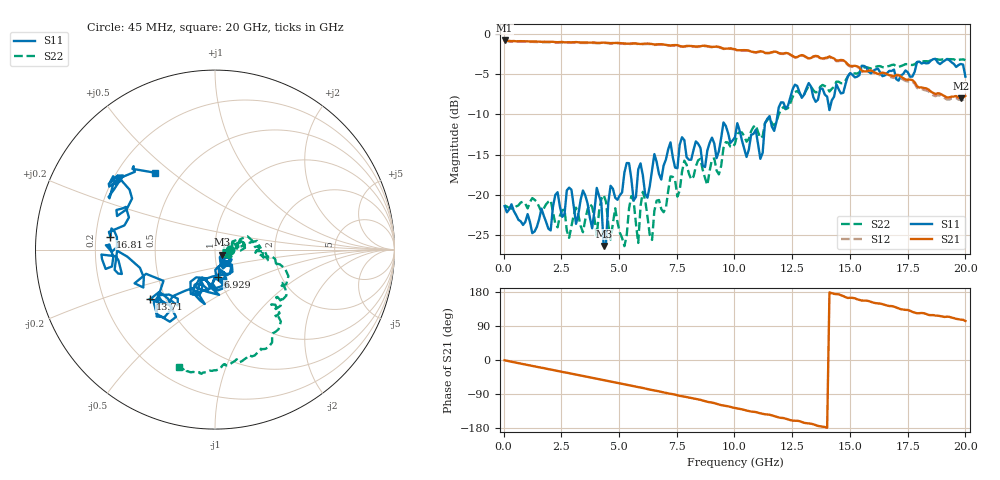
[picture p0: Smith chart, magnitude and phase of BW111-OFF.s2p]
!  2-Port S-parameters saved by WinCal
! VAR MeasName=S-Parameters (CALIBRATED_DATA) read from VNA (E8364A)
! VAR MeasDate=10/28/2010 3:35:15 PM
! VAR NAME=5-1you 2
! VAR FILENAME=5-1you 2.s2p
! VAR DATE=10/28/2010 3:35:15 PM
! VAR PHYS_PORTS=1,2
# Hz S RI R 50
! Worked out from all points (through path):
!   201 points, 45 MHz to 20 GHz, reference 50 ohm
!   highest |S21| = -0.83 dB at 45 MHz (marker M1); lowest = -8.0 dB at 19.8 GHz (marker M2)
!   group delay of S21, straight-line fit = 36.3 ps
!   lowest |S11| = -26.3 dB at 4.335 GHz (marker M3), VSWR 1.10, Z = 54 - j3.04 ohm
!   |S11| at or under -10 dB: start of sweep to 11.87 GHz
!   |S22| runs from -26.4 to -3.1 dB; largest |S21 - S12| = 0.015
!   S11 on the Smith chart (normalised r, x): 45 MHz: 1.19, -0.01; 6.929 GHz: 0.99, -0.30; 13.71 GHz: 0.41, -0.29; 16.81 GHz: 0.26, +0.06; 20 GHz: 0.36, +0.44
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4.5e7  0.0851 -0.00237  0.9088 -0.00982  0.9029 -0.011  0.086 -0.00114
3.43735e9  0.0763 -0.0743  0.6546 -0.5912  0.6508 -0.5872  0.0572 -0.0129
3.83645e9  0.0364 -0.0502  0.601 -0.646  0.5977 -0.642  0.0757 -0.0371
4.036e9  0.0659 -0.0886  0.5725 -0.6662  0.5683 -0.6625  0.0537 -0.0147
4.335325e9  0.0391 -0.0281  0.5285 -0.7057  0.5245 -0.7014  0.0917 -0.0395
4.63465e9  0.0446 -0.1047  0.479 -0.7324  0.4759 -0.7266  0.0479 -0.0224
5.333075e9  0.069 -0.1418  0.3619 -0.7891  0.3587 -0.7826  0.054 0.0156
5.6324e9  0.06 -0.0703  0.3125 -0.8147  0.3113 -0.8099  0.0897 -0.0189
5.83195e9  0.0288 -0.1412  0.2728 -0.8222  0.271 -0.8189  0.0502 0.00282
6.0315e9  0.0912 -0.0957  0.2413 -0.8324  0.2392 -0.8271  0.1044 0.0031
6.4306e9  0.00617 -0.1429  0.16 -0.8482  0.1578 -0.8422  0.0523 0.00395
6.729925e9  0.049 -0.1257  0.1099 -0.8542  0.1096 -0.85  0.0928 0.00622
6.929475e9  0.0157 -0.151  0.0667 -0.8548  0.067 -0.8499  0.0767 0.0145
1.00225e10  -0.1142 -0.1972  -0.4801 -0.6427  -0.4778 -0.6393  0.2036 0.0418
1.112002e10  -0.0524 -0.1591  -0.6024 -0.4938  -0.5993 -0.4885  0.2244 -0.0164
1.261665e10  -0.3238 -0.3586  -0.6734 -0.2414  -0.6725 -0.2333  0.409 -0.1474
1.341485e10  -0.2386 -0.3258  -0.7115 -0.1305  -0.7071 -0.1265  0.3496 -0.2775
1.371418e10  -0.363 -0.2773  -0.7032 -0.0615  -0.6992 -0.054  0.3696 -0.2888
1.670742e10  -0.5767 0.1178  -0.4381 0.3371  -0.4251 0.335  0.167 -0.6091
1.68072e10  -0.583 0.0722  -0.4343 0.336  -0.4224 0.3308  0.1483 -0.6226
1.980045e10  -0.454 0.4648  -0.1136 0.3821  -0.1126 0.3721  -0.1864 -0.6666
2e10  -0.3321 0.428  -0.0924 0.4008  -0.0938 0.39  -0.2029 -0.6555
